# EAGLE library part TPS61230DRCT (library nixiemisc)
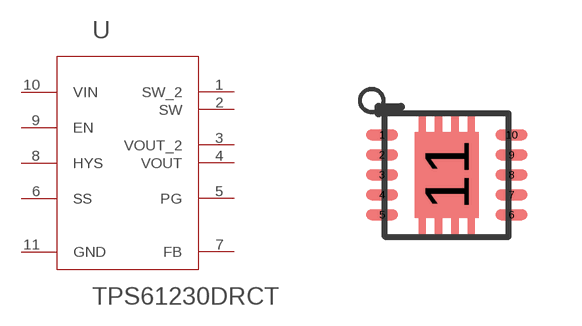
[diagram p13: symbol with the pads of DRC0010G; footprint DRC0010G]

Designator prefix U

## TPS61230DRCT  [DRC0010G]
1  SW_2  pwr
2  SW  pwr
3  VOUT_2  pwr
4  VOUT  pwr
5  PG  out
6  SS  in
7  FB  in
8  HYS  out
9  EN  in
10  VIN  pwr
11  GND  pwr

## Footprint DRC0010G (pad centres in mm)
smd 0.8 x 0.28: 1 -1.62,1; 2 -1.62,0.5; 3 -1.62,0; 4 -1.62,-0.5; 5 -1.62,-1; 6 1.62,-1; 7 1.62,-0.5; 8 1.62,0; 9 1.62,0.5; 10 1.62,1
smd 1.6 x 2.15: 11 0,0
